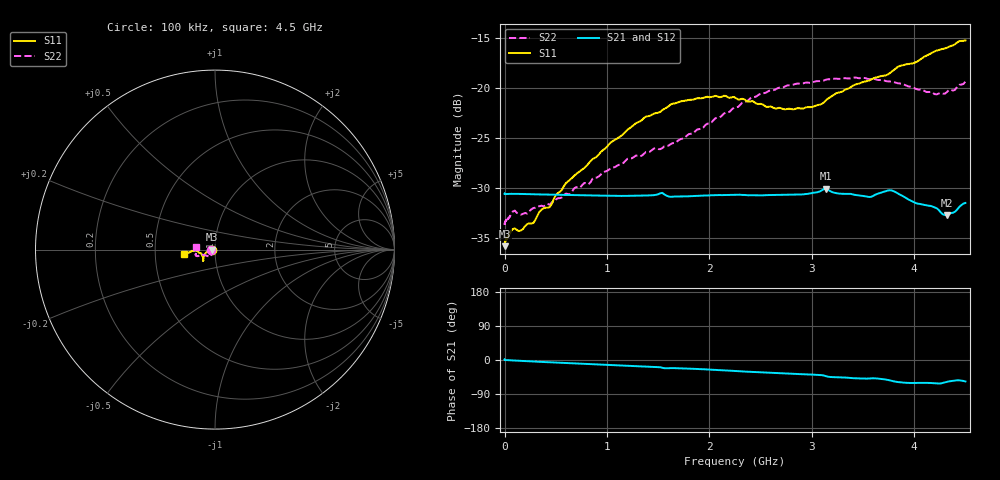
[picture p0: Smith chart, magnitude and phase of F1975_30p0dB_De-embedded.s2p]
! Integrated Device Technology
! Corporate Headquarters
! 6024 Silver Creek Valley Road
! San Jose, CA 95138  USA
! Phone:  1-408-284-8200
! Toll Free:  1-800-223-1366
! Webpage:  http://www.idt.com/
! Timing and RF Division
! 515 Groton Road, Suite 102
! Westford, MA 01886-6024
! Device:  F1975
! Description: 6-bit, 75 ohm, 0.5 dB Digital Step Attenuator
! Frequency:  5.0 MHz -  3.00 GHz
! Package:  4x4 mm QFN Plastic Package: 20 pin
! Ports:  2 RF, 11 DC
!  Pin  1  = D5 (16 dB)
!  Pin  2  = RF1  =  Port 1
!  Pin  3  = Serial Data In (DATA)
!  Pin  4  = Serial Clock (CLK)
!  Pin  5  = Serial Latch Enable (LE)
!  Pin  6  = VDD
!  Pin  7  = NC
!  Pin  8  = NC
!  Pin  9  = NC
!  Pin 10  = GND
!  Pin 11  = GND
!  Pin 12  = NC
!  Pin 13  = VMODE
!  Pin 14  = RF2  =  Port 2
!  Pin 15  = D4 (8 dB)
!  Pin 16  = D3 (4 dB)
!  Pin 17  = D2 (2 dB)
!  Pin 18  = NC
!  Pin 19  = D1 (1 dB)
!  Pin 20  = D0 (0.5 dB)
! State:  60
! Atten State:  30.0 dB
! Voltage:  +3.30 Volts
! Current:  0.591 mA
! Data:  The device was measured on a F1975 evaluation board which has
!  individual transmission lines to the RF pins.  Data was collected
!  using a calibrated network analyzer.  The evaluation board was
!  de-embedded using Automatic Fixture Removal (AFR).
!  The reference plane is the edge of the package pin.
! Misc:
!  Action Tracker AT0415
! Date Measured:  2018-02-08
! Date:  2018-03-26  MJV
! Note:
!  Integrated Device Technology supplies this data as a sample of measured
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# GHz S dB R 75
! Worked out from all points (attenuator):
!   291 points, 100 kHz to 4.5 GHz, reference 75 ohm
!   highest |S21| = -30.09 dB at 3.14 GHz (marker M1); lowest = -32.7 dB at 4.32 GHz (marker M2)
!   lowest |S11| = -35.8 dB at 300 kHz (marker M3), VSWR 1.03, Z = 72.6 - j0.0411 ohm
!   |S11| at or under -10 dB: start of sweep to end of sweep
!   |S22| runs from -33.7 to -19.0 dB; largest |S21 - S12| = 0.00016
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0.0001  -35.84 179.7  -30.59 1.2  -30.57 1.2  -33.73 -178.8
0.0003  -35.85 -179.0  -30.59 1.1  -30.56 1.1  -33.63 -178.6
0.005  -35.32 -178.2  -30.62 0.6  -30.62 0.6  -33.44 -177.3
0.08  -34.14 -176.2  -30.61 -1.1  -30.61 -1.1  -32.38 -169.6
0.16  -34.28 -177.0  -30.63 -2.3  -30.63 -2.3  -32.69 -160.1
0.28  -33.53 179.7  -30.65 -4.0  -30.65 -4.0  -32.04 -152.0
0.36  -32.19 -179.9  -30.67 -5.0  -30.67 -5.0  -31.80 -144.5
0.44  -31.94 -179.3  -30.69 -6.1  -30.69 -6.1  -31.70 -139.0
0.6  -29.53 -175.7  -30.73 -8.1  -30.73 -8.1  -30.59 -133.1
0.76  -28.18 -169.0  -30.76 -10.1  -30.76 -10.1  -29.70 -129.2
1.28  -23.56 -152.9  -30.80 -16.2  -30.80 -16.1  -26.80 -124.8
1.52  -22.42 -145.8  -30.56 -19.1  -30.55 -19.1  -26.14 -131.3
1.88  -21.05 -139.1  -30.82 -23.7  -30.82 -23.7  -24.19 -147.2
2.26  -21.04 -137.8  -30.71 -29.1  -30.71 -29.1  -21.95 -157.9
2.64  -22.07 -148.0  -30.73 -34.2  -30.73 -34.2  -20.20 -159.4
3.02  -21.88 -164.7  -30.50 -38.9  -30.49 -38.9  -19.42 -160.2
3.14  -21.24 -167.3  -30.09 -42.9  -30.09 -42.9  -19.19 -160.6
3.56  -19.28 -177.6  -30.93 -48.9  -30.93 -48.9  -19.15 -166.1
3.76  -18.56 -176.2  -30.26 -53.6  -30.25 -53.6  -19.37 -169.8
4.2  -16.37 -173.2  -31.97 -61.3  -31.96 -61.3  -20.64 178.6
4.32  -16.00 -172.6  -32.73 -57.5  -32.73 -57.5  -20.43 176.1
4.5  -15.27 -172.3  -31.52 -56.6  -31.52 -56.6  -19.39 173.5
